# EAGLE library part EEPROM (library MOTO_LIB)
I2C EE PROM, 8 pin
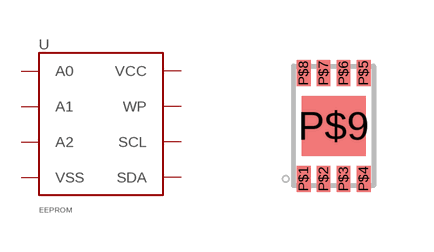
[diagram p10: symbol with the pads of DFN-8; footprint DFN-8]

Designator prefix -

## EEPROMDFN8 (MPN: BR24G16NUX-3; SUPPLIER: ROHM)  [DFN-8]
P$1  A0  in
P$2  A1  in
P$3  A2  in
P$4  VSS  pwr
P$5  SDA
P$6  SCL  in
P$7  WP  in
P$8  VCC  pwr
P$9  VSS  pwr

## Footprint DFN-8 (pad centres in mm)
Now follows http://pdfserv.maximintegrated.com/land_patterns/90-0065.PDF Pasted was reduced by 40% width on the center ground pad, and some amount on the other 8. Stop mask extends 135 µm wider than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
smd 0.35 x 0.65: P$1 -0.75,-1.325; P$2 -0.25,-1.325; P$3 0.25,-1.325; P$4 0.75,-1.325; P$5 0.75,1.325; P$6 0.25,1.325; P$7 -0.25,1.325; P$8 -0.75,1.325
smd 1.6 x 1.5: P$9 0,0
